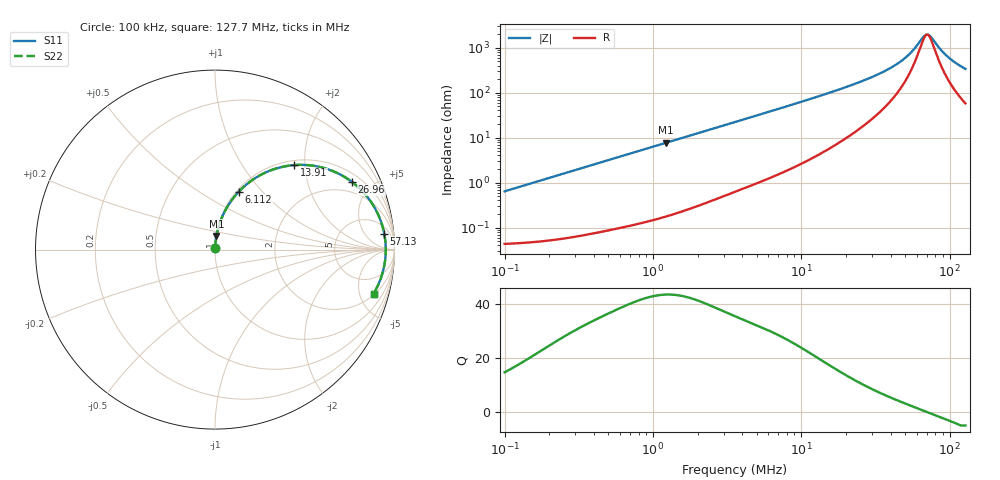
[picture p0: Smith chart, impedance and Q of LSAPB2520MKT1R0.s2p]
! LSAPB2520MKT1R0  S-PARAMETER MODEL  ( General Type )
! Model Generated by TAIYO YUDEN Corporation (http://www.ty-top.com)
! Version 2.0
! TAIYO YUDEN Control No. 20210629
! Copyright(c) 2015 TAIYO YUDEN CO.,LTD. All Rights Reserved.
! Product Description (link to TY-COMPAS)
! https://ds.yuden.co.jp/TYCOMPAS/or/detail?pn=LSAPB2520MKT1R0M&u=M
! Products Name : Inductors
! Characteristics :
!  Inductance : 1.0 uH , SRF(min) : -Hz , DC Resistance(max) : 0.045 Ohm
!  Rated Current : Saturation :4300 mA , Temp Rise : 3100 mA (40 degC)
!  Case Size : 2.5 x 2.0 / 0.098 x 0.079 [mm/inch] , Thickness : 1.2 / 0.047 [mm/inch]
!  (Conditions: Temperature = 25 degC , DC Bias Current/Voltage = 0A / 0V)
! External Node Assignments :
!  1  o---GGG---o  2
! GND o---------o GND
! Frequency Range : 0.1MHz  -  127.746476MHz  [ 402 STEP ]
# MHz S RI R 50
! Freq[MHz].  S11 Real  S11 Imag  S21 Real  S21 Imag  S12 Real  S12 Imag  S22 Real  S22 Imag
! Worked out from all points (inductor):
!   401 points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, 100 kHz to 127.7 MHz, reference 50 ohm
!   read as one part in series: L = 1.01 uH near 103.6 kHz
!   highest Q = 43.6 at 1.222 MHz (marker M1), where L = 995 nH
!   self-resonance near 70.54 MHz
!   S11 on the Smith chart (normalised r, x): 100 kHz: 1.00, +0.01; 6.112 MHz: 1.03, +0.76; 13.91 MHz: 1.09, +1.76; 26.96 MHz: 1.39, +3.81; 57.13 MHz: 9, +16; 127.7 MHz: 2.15, -6.63
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0.1  0.000473 0.00637  0.9995 -0.00637  0.9995 -0.00637  0.000473 0.00637
0.33137  0.0011 0.021  0.9989 -0.021  0.9989 -0.021  0.0011 0.021
1.098062  0.00626 0.0682  0.9937 -0.0682  0.9937 -0.0682  0.00626 0.0682
1.222425  0.00753 0.0757  0.9925 -0.0757  0.9925 -0.0757  0.00753 0.0757
3.574164  0.0521 0.2086  0.9479 -0.2086  0.9479 -0.2086  0.0521 0.2086
6.11154  0.1331 0.3235  0.8669 -0.3235  0.8669 -0.3235  0.1331 0.3235
8.432111  0.2238 0.3982  0.7762 -0.3982  0.7762 -0.3982  0.2238 0.3982
11.84371  0.3626 0.4579  0.6374 -0.4579  0.6374 -0.4579  0.3626 0.4579
13.91172  0.4412 0.4709  0.5588 -0.4709  0.5588 -0.4709  0.4412 0.4709
19.19404  0.6071 0.4546  0.3929 -0.4546  0.3929 -0.4546  0.6071 0.4546
26.95988  0.7639 0.3766  0.2361 -0.3766  0.2361 -0.3766  0.7639 0.3766
39.24654  0.8842 0.2425  0.1158 -0.2425  0.1158 -0.2425  0.8842 0.2425
48.63981  0.9249 0.1556  0.0751 -0.1556  0.0751 -0.1556  0.9249 0.1556
57.13269  0.943 0.0886  0.057 -0.0886  0.057 -0.0886  0.943 0.0886
67.1085  0.951 0.021  0.049 -0.021  0.049 -0.021  0.951 0.021
69.55194  0.9514 0.00594  0.0486 -0.00594  0.0486 -0.00594  0.9514 0.00594
72.08436  0.9514 -0.00911  0.0486 0.00911  0.0486 0.00911  0.9514 -0.00911
74.70897  0.9509 -0.0242  0.0491 0.0242  0.0491 0.0242  0.9509 -0.0242
86.19851  0.944 -0.0843  0.056 0.0843  0.056 0.0843  0.944 -0.0843
95.96105  0.9337 -0.1292  0.0663 0.1292  0.0663 0.1292  0.9337 -0.1292
110.7189  0.9128 -0.1883  0.0872 0.1883  0.0872 0.1883  0.9128 -0.1883
127.7465  0.8832 -0.246  0.1168 0.246  0.1168 0.246  0.8832 -0.246
